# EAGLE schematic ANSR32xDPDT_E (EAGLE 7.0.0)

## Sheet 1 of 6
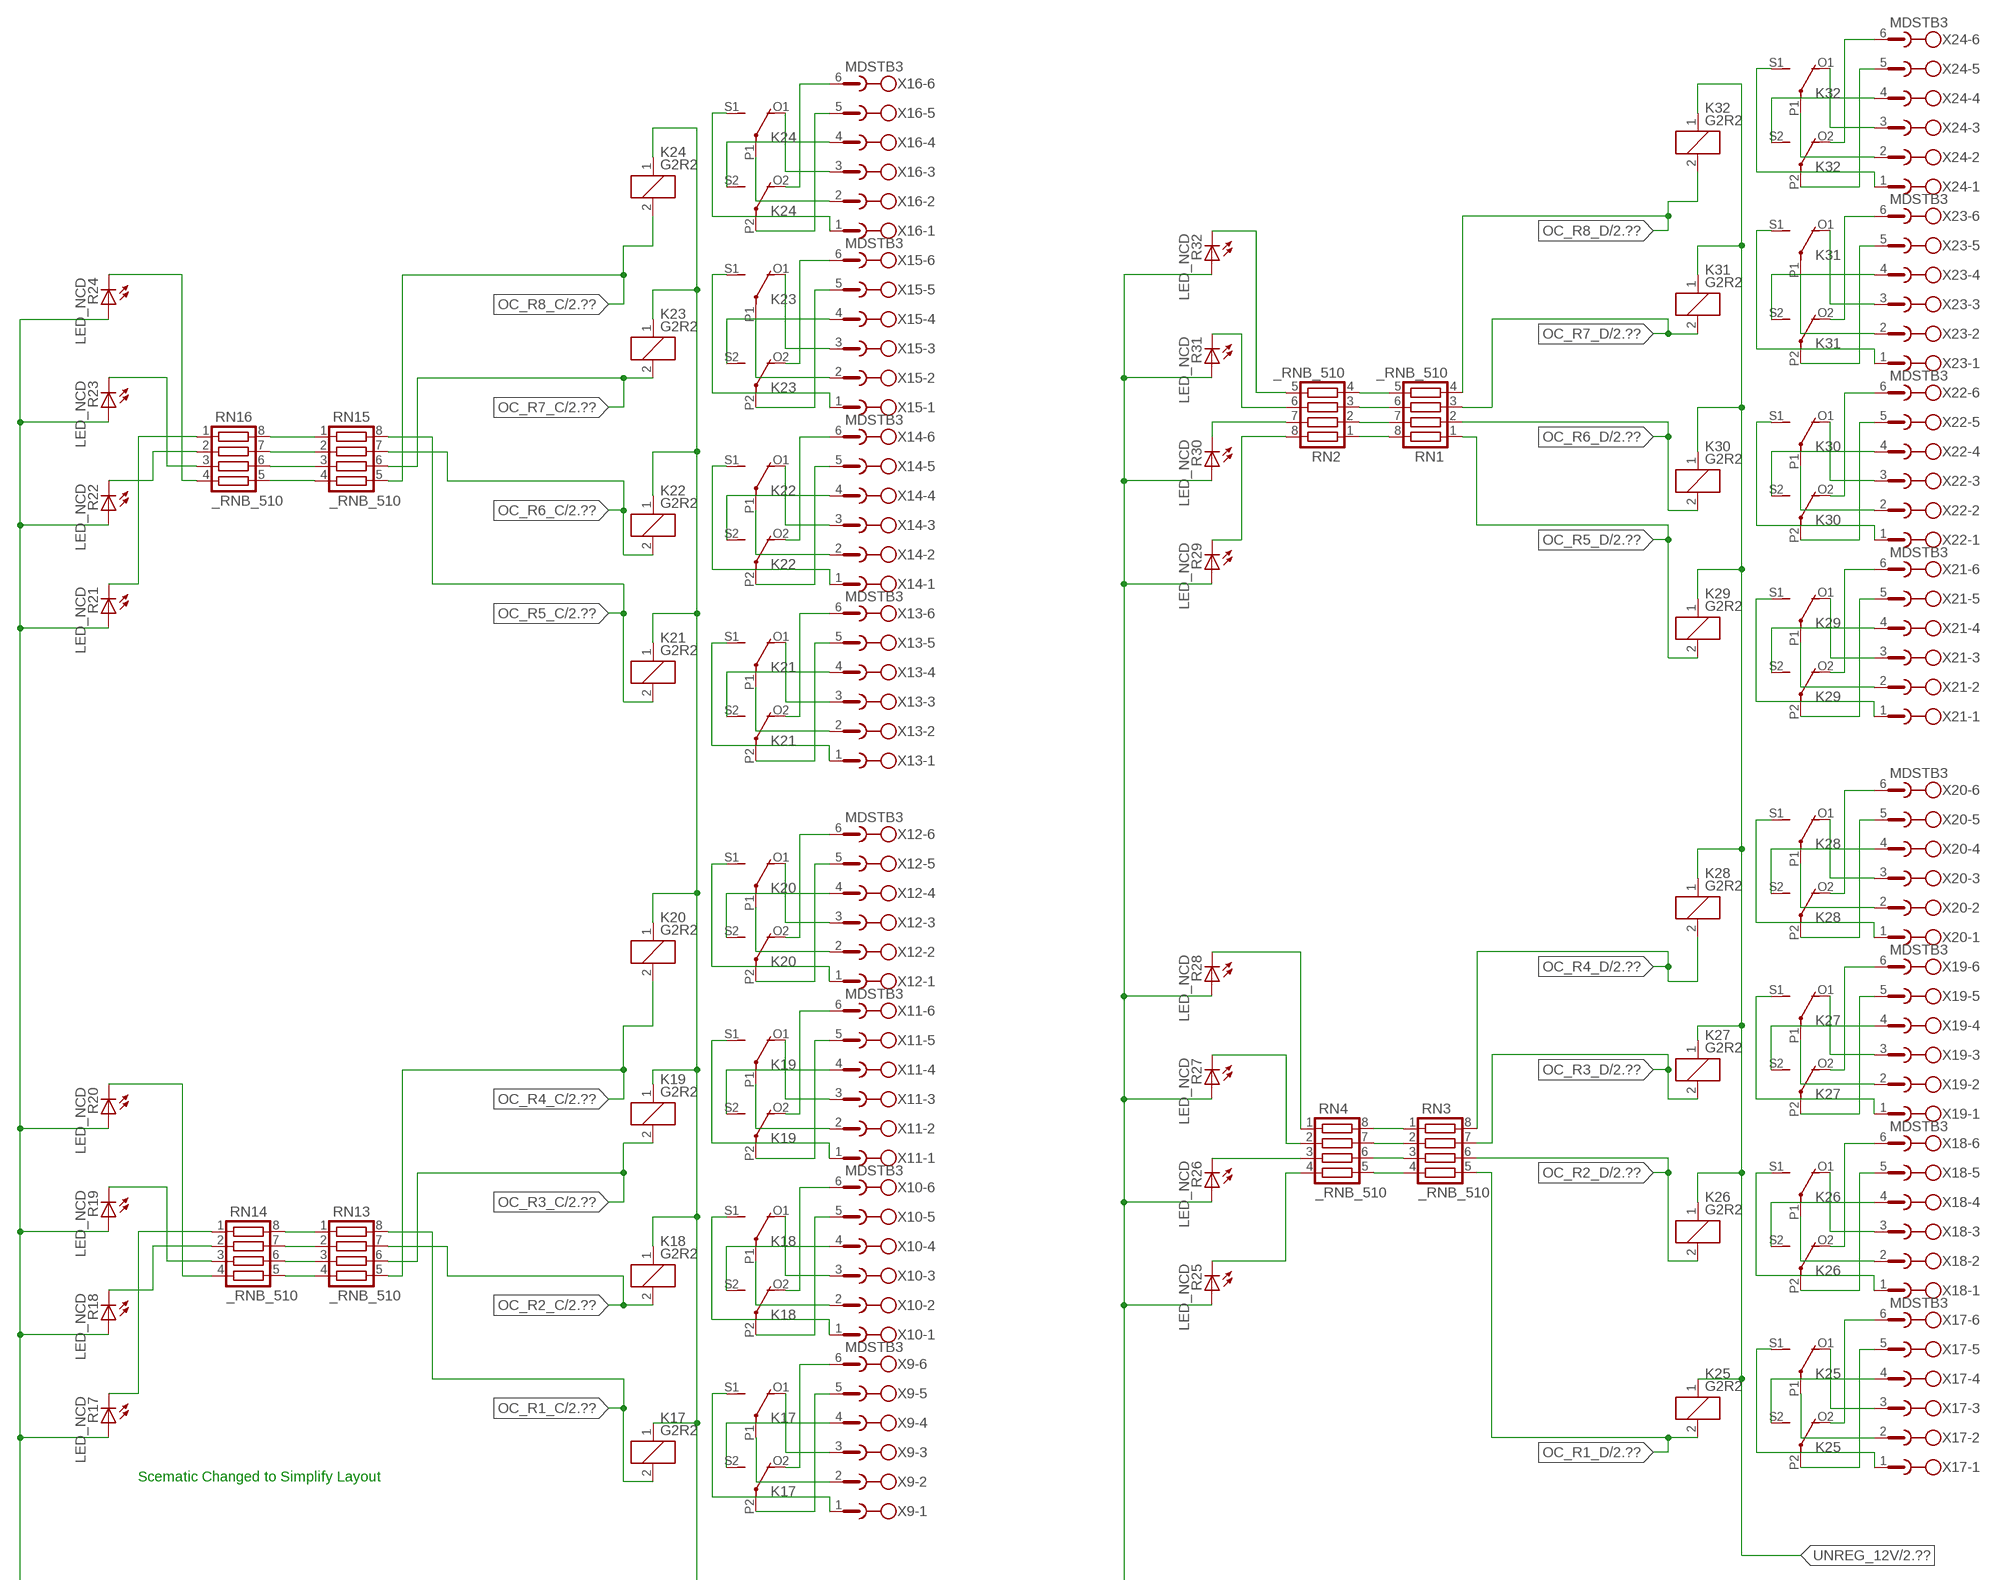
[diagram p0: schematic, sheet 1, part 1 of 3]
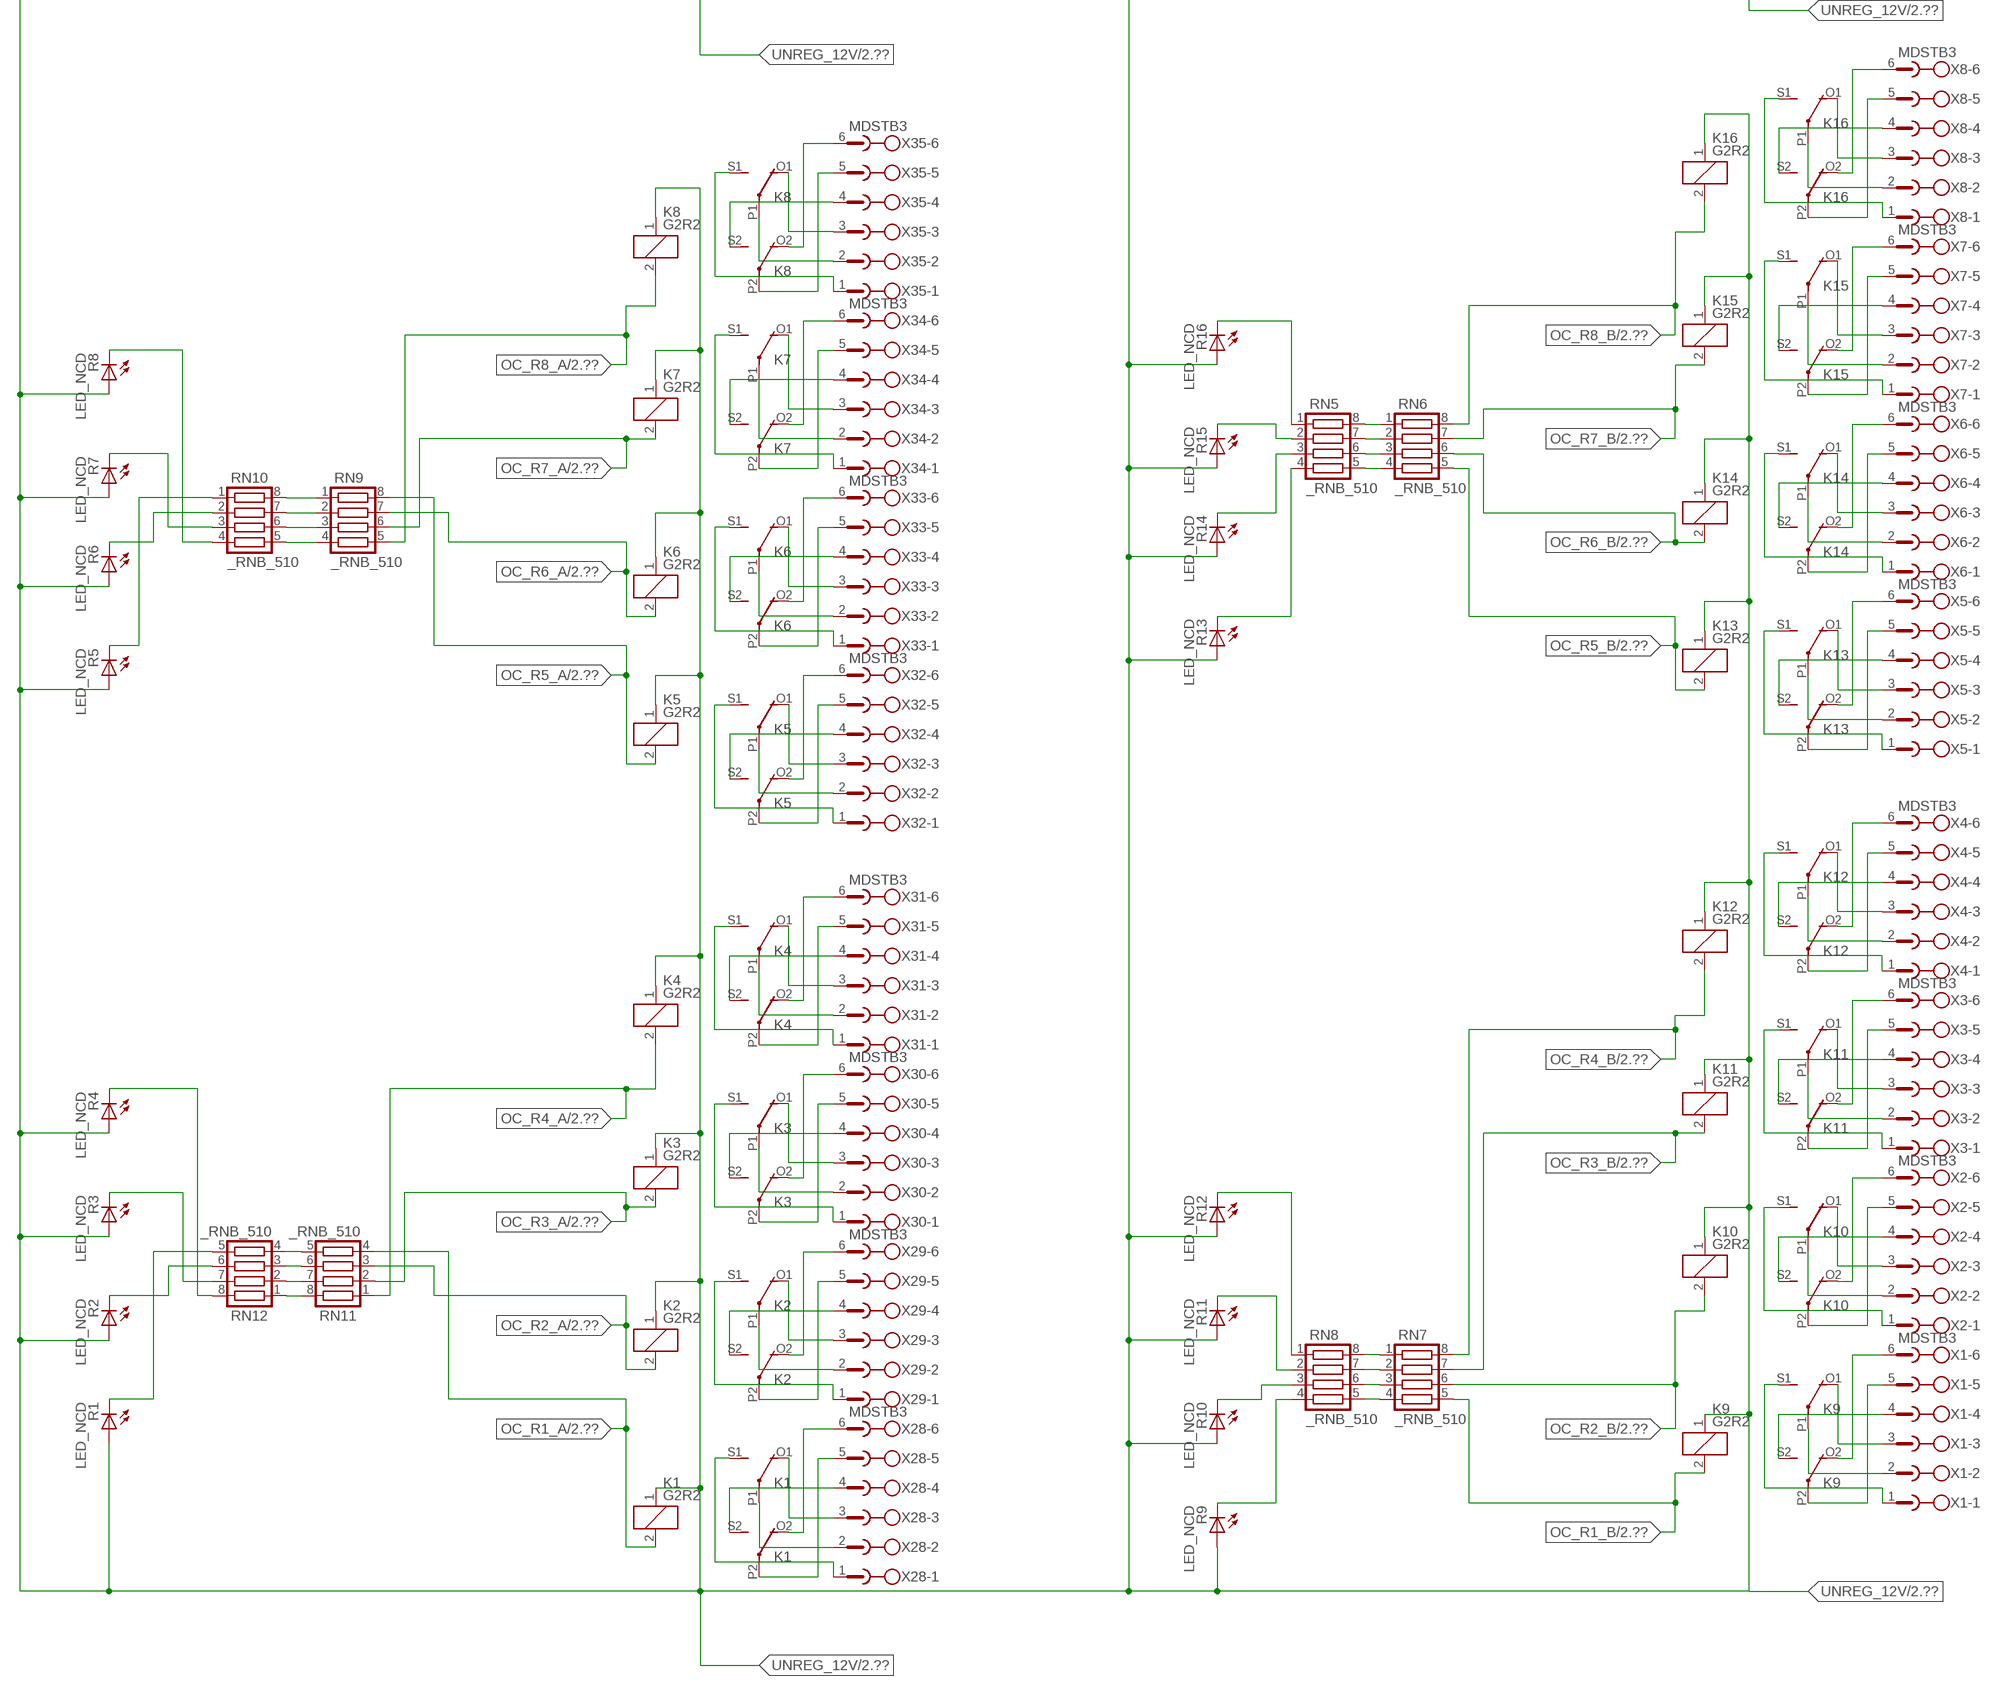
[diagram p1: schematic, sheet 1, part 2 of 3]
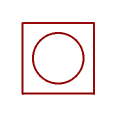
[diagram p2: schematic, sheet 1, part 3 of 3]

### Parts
K1  G2R2  [G2R2]
K2  G2R2  [G2R2]
K3  G2R2  [G2R2]
K4  G2R2  [G2R2]
K5  G2R2  [G2R2]
K6  G2R2  [G2R2]
K7  G2R2  [G2R2]
K8  G2R2  [G2R2]
K9  G2R2  [G2R2]
K10  G2R2  [G2R2]
K11  G2R2  [G2R2]
K12  G2R2  [G2R2]
K13  G2R2  [G2R2]
K14  G2R2  [G2R2]
K15  G2R2  [G2R2]
K16  G2R2  [G2R2]
K17  G2R2  [G2R2]
K18  G2R2  [G2R2]
K19  G2R2  [G2R2]
K20  G2R2  [G2R2]
K21  G2R2  [G2R2]
K22  G2R2  [G2R2]
K23  G2R2  [G2R2]
K24  G2R2  [G2R2]
K25  G2R2  [G2R2]
K26  G2R2  [G2R2]
K27  G2R2  [G2R2]
K28  G2R2  [G2R2]
K29  G2R2  [G2R2]
K30  G2R2  [G2R2]
K31  G2R2  [G2R2]
K32  G2R2  [G2R2]
R1  LED_NCD  [CHIPLED_0603]
R2  LED_NCD  [CHIPLED_0603]
R3  LED_NCD  [CHIPLED_0603]
R4  LED_NCD  [CHIPLED_0603]
R5  LED_NCD  [CHIPLED_0603]
R6  LED_NCD  [CHIPLED_0603]
R7  LED_NCD  [CHIPLED_0603]
R8  LED_NCD  [CHIPLED_0603]
R9  LED_NCD  [CHIPLED_0603]
R10  LED_NCD  [CHIPLED_0603]
R11  LED_NCD  [CHIPLED_0603]
R12  LED_NCD  [CHIPLED_0603]
R13  LED_NCD  [CHIPLED_0603]
R14  LED_NCD  [CHIPLED_0603]
R15  LED_NCD  [CHIPLED_0603]
R16  LED_NCD  [CHIPLED_0603]
R17  LED_NCD  [CHIPLED_0603]
R18  LED_NCD  [CHIPLED_0603]
R19  LED_NCD  [CHIPLED_0603]
R20  LED_NCD  [CHIPLED_0603]
R21  LED_NCD  [CHIPLED_0603]
R22  LED_NCD  [CHIPLED_0603]
R23  LED_NCD  [CHIPLED_0603]
R24  LED_NCD  [CHIPLED_0603]
R25  LED_NCD  [CHIPLED_0603]
R26  LED_NCD  [CHIPLED_0603]
R27  LED_NCD  [CHIPLED_0603]
R28  LED_NCD  [CHIPLED_0603]
R29  LED_NCD  [CHIPLED_0603]
R30  LED_NCD  [CHIPLED_0603]
R31  LED_NCD  [CHIPLED_0603]
R32  LED_NCD  [CHIPLED_0603]
RN1  _RNB_510  [RNB]
RN2  _RNB_510  [RNB]
RN3  _RNB_510  [RNB]
RN4  _RNB_510  [RNB]
RN5  _RNB_510  [RNB]
RN6  _RNB_510  [RNB]
RN7  _RNB_510  [RNB]
RN8  _RNB_510  [RNB]
RN9  _RNB_510  [RNB]
RN10  _RNB_510  [RNB]
RN11  _RNB_510  [RNB]
RN12  _RNB_510  [RNB]
RN13  _RNB_510  [RNB]
RN14  _RNB_510  [RNB]
RN15  _RNB_510  [RNB]
RN16  _RNB_510  [RNB]
U$1  PCB_MOUNTING_HOLE  [PCB_MOUNTING_HOLE]
X1  MDSTB3  [MDSTB3]
X2  MDSTB3  [MDSTB3]
X3  MDSTB3  [MDSTB3]
X4  MDSTB3  [MDSTB3]
X5  MDSTB3  [MDSTB3]
X6  MDSTB3  [MDSTB3]
X7  MDSTB3  [MDSTB3]
X8  MDSTB3  [MDSTB3]
X9  MDSTB3  [MDSTB3]
X10  MDSTB3  [MDSTB3]
X11  MDSTB3  [MDSTB3]
X12  MDSTB3  [MDSTB3]
X13  MDSTB3  [MDSTB3]
X14  MDSTB3  [MDSTB3]
X15  MDSTB3  [MDSTB3]
X16  MDSTB3  [MDSTB3]
X17  MDSTB3  [MDSTB3]
X18  MDSTB3  [MDSTB3]
X19  MDSTB3  [MDSTB3]
X20  MDSTB3  [MDSTB3]
X21  MDSTB3  [MDSTB3]
X22  MDSTB3  [MDSTB3]
X23  MDSTB3  [MDSTB3]
X24  MDSTB3  [MDSTB3]
X28  MDSTB3  [MDSTB3]
X29  MDSTB3  [MDSTB3]
X30  MDSTB3  [MDSTB3]
X31  MDSTB3  [MDSTB3]
X32  MDSTB3  [MDSTB3]
X33  MDSTB3  [MDSTB3]
X34  MDSTB3  [MDSTB3]
X35  MDSTB3  [MDSTB3]

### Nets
N$1: K9.P2(3:COM) X1.5
N$2: K9.O2(3:NC) X1.6
N$3: K9.S2(3:NO) X1.4
N$4: K9.P1(2:COM) X1.2
N$5: K9.O1(2:NC) X1.3
N$6: K9.S1(2:NO) X1.1
N$7: K10.P2(3:COM) X2.5
N$8: K10.O2(3:NC) X2.6
N$9: K10.S2(3:NO) X2.4
N$10: K10.S1(2:NO) X2.1
N$11: K10.P1(2:COM) X2.2
N$12: K10.O1(2:NC) X2.3
N$13: K11.P2(3:COM) X3.5
N$14: K11.O2(3:NC) X3.6
N$15: K12.P2(3:COM) X4.5
N$16: K12.O2(3:NC) X4.6
N$17: K11.S2(3:NO) X3.4
N$18: K12.S2(3:NO) X4.4
N$19: K11.O1(2:NC) X3.3
N$20: K12.O1(2:NC) X4.3
N$21: K12.P1(2:COM) X4.2
N$22: K11.P1(2:COM) X3.2
N$23: K11.S1(2:NO) X3.1
N$24: K12.S1(2:NO) X4.1
N$25: K13.O2(3:NC) X5.6
N$26: K13.P2(3:COM) X5.5
N$27: K13.S2(3:NO) X5.4
N$28: K13.P1(2:COM) X5.2
N$29: K13.S1(2:NO) X5.1
N$30: K13.O1(2:NC) X5.3
N$31: K14.P2(3:COM) X6.5
N$32: K14.O2(3:NC) X6.6
N$33: K14.P1(2:COM) X6.2
N$34: K14.S1(2:NO) X6.1
N$35: K15.P1(2:COM) X7.2
N$36: K16.P1(2:COM) X8.2
N$37: K16.P2(3:COM) X8.5
N$38: K16.O2(3:NC) X8.6
N$39: K14.O1(2:NC) X6.3
N$40: K16.O1(2:NC) X8.3
N$41: K15.O1(2:NC) X7.3
N$42: K15.O2(3:NC) X7.6
N$43: K15.P2(3:COM) X7.5
N$44: K14.S2(3:NO) X6.4
N$45: K15.S2(3:NO) X7.4
N$46: K15.S1(2:NO) X7.1
N$47: K16.S1(2:NO) X8.1
N$48: K16.S2(3:NO) X8.4
N$49: K17.P2(3:COM) X9.5
N$50: K17.O2(3:NC) X9.6
N$51: K17.S2(3:NO) X9.4
N$52: K17.P1(2:COM) X9.2
N$53: K17.O1(2:NC) X9.3
N$54: K17.S1(2:NO) X9.1
N$55: K18.P2(3:COM) X10.5
N$56: K18.O2(3:NC) X10.6
N$57: K18.S2(3:NO) X10.4
N$58: K18.S1(2:NO) X10.1
N$59: K18.P1(2:COM) X10.2
N$60: K18.O1(2:NC) X10.3
N$61: K19.P2(3:COM) X11.5
N$62: K19.O2(3:NC) X11.6
N$63: K20.P2(3:COM) X12.5
N$64: K20.O2(3:NC) X12.6
N$65: K19.S2(3:NO) X11.4
N$66: K20.S2(3:NO) X12.4
N$67: K19.O1(2:NC) X11.3
N$68: K20.O1(2:NC) X12.3
N$69: K20.P1(2:COM) X12.2
N$70: K19.P1(2:COM) X11.2
N$71: K19.S1(2:NO) X11.1
N$72: K20.S1(2:NO) X12.1
N$73: K21.O2(3:NC) X13.6
N$74: K21.P2(3:COM) X13.5
N$75: K21.S2(3:NO) X13.4
N$76: K21.P1(2:COM) X13.2
N$77: K21.S1(2:NO) X13.1
N$78: K21.O1(2:NC) X13.3
N$79: K22.P2(3:COM) X14.5
N$80: K22.O2(3:NC) X14.6
N$81: K22.P1(2:COM) X14.2
N$82: K22.S1(2:NO) X14.1
N$83: K23.P1(2:COM) X15.2
N$84: K24.P1(2:COM) X16.2
N$85: K24.P2(3:COM) X16.5
N$86: K24.O2(3:NC) X16.6
N$87: K22.O1(2:NC) X14.3
N$88: K24.O1(2:NC) X16.3
N$89: K23.O1(2:NC) X15.3
N$90: K23.O2(3:NC) X15.6
N$91: K23.P2(3:COM) X15.5
N$92: K22.S2(3:NO) X14.4
N$93: K23.S2(3:NO) X15.4
N$94: K23.S1(2:NO) X15.1
N$95: K24.S1(2:NO) X16.1
N$96: K24.S2(3:NO) X16.4
N$97: K25.P2(3:COM) X17.5
N$98: K25.O2(3:NC) X17.6
N$99: K25.S2(3:NO) X17.4
N$100: K25.P1(2:COM) X17.2
N$101: K25.O1(2:NC) X17.3
N$102: K25.S1(2:NO) X17.1
N$103: K26.P2(3:COM) X18.5
N$104: K26.O2(3:NC) X18.6
N$105: K26.S2(3:NO) X18.4
N$106: K26.S1(2:NO) X18.1
N$107: K26.P1(2:COM) X18.2
N$108: K26.O1(2:NC) X18.3
N$109: K27.P2(3:COM) X19.5
N$110: K27.O2(3:NC) X19.6
N$111: K28.P2(3:COM) X20.5
N$112: K28.O2(3:NC) X20.6
N$113: K27.S2(3:NO) X19.4
N$114: K28.S2(3:NO) X20.4
N$115: K27.O1(2:NC) X19.3
N$116: K28.O1(2:NC) X20.3
N$117: K28.P1(2:COM) X20.2
N$118: K27.P1(2:COM) X19.2
N$119: K27.S1(2:NO) X19.1
N$120: K28.S1(2:NO) X20.1
N$121: K29.O2(3:NC) X21.6
N$122: K29.P2(3:COM) X21.5
N$123: K29.S2(3:NO) X21.4
N$124: K29.P1(2:COM) X21.2
N$125: K29.S1(2:NO) X21.1
N$126: K29.O1(2:NC) X21.3
N$127: K30.P2(3:COM) X22.5
N$128: K30.O2(3:NC) X22.6
N$129: K30.P1(2:COM) X22.2
N$130: K30.S1(2:NO) X22.1
N$131: K31.P1(2:COM) X23.2
N$132: K32.P1(2:COM) X24.2
N$133: K32.P2(3:COM) X24.5
N$134: K32.O2(3:NC) X24.6
N$135: K30.O1(2:NC) X22.3
N$136: K32.O1(2:NC) X24.3
N$137: K31.O1(2:NC) X23.3
N$138: K31.O2(3:NC) X23.6
N$139: K31.P2(3:COM) X23.5
N$140: K30.S2(3:NO) X22.4
N$141: K31.S2(3:NO) X23.4
N$142: K31.S1(2:NO) X23.1
N$143: K32.S1(2:NO) X24.1
N$144: K32.S2(3:NO) X24.4
N$203: K1.P2(3:COM) X28.5
N$204: K1.O2(3:NC) X28.6
N$205: K1.S2(3:NO) X28.4
N$206: K1.P1(2:COM) X28.2
N$207: K1.O1(2:NC) X28.3
N$208: K1.S1(2:NO) X28.1
N$209: K2.P2(3:COM) X29.5
N$210: K2.O2(3:NC) X29.6
N$211: K2.S2(3:NO) X29.4
N$212: K2.S1(2:NO) X29.1
N$213: K2.P1(2:COM) X29.2
N$214: K2.O1(2:NC) X29.3
N$215: K3.P2(3:COM) X30.5
N$216: K3.O2(3:NC) X30.6
N$217: K4.P2(3:COM) X31.5
N$218: K4.O2(3:NC) X31.6
N$219: K3.S2(3:NO) X30.4
N$220: K4.S2(3:NO) X31.4
N$221: K3.O1(2:NC) X30.3
N$222: K4.O1(2:NC) X31.3
N$223: K4.P1(2:COM) X31.2
N$224: K3.P1(2:COM) X30.2
N$225: K3.S1(2:NO) X30.1
N$226: K4.S1(2:NO) X31.1
N$304: K5.O2(3:NC) X32.6
N$305: K5.P2(3:COM) X32.5
N$306: K5.S2(3:NO) X32.4
N$307: K5.P1(2:COM) X32.2
N$308: K5.S1(2:NO) X32.1
N$309: K5.O1(2:NC) X32.3
N$310: K6.P2(3:COM) X33.5
N$311: K6.O2(3:NC) X33.6
N$312: K6.P1(2:COM) X33.2
N$313: K6.S1(2:NO) X33.1
N$314: K7.P1(2:COM) X34.2
N$315: K8.P1(2:COM) X35.2
N$316: K8.P2(3:COM) X35.5
N$317: K8.O2(3:NC) X35.6
N$318: K6.O1(2:NC) X33.3
N$319: K8.O1(2:NC) X35.3
N$320: K7.O1(2:NC) X34.3
N$321: K7.O2(3:NC) X34.6
N$322: K7.P2(3:COM) X34.5
N$323: K6.S2(3:NO) X33.4
N$324: K7.S2(3:NO) X34.4
N$325: K7.S1(2:NO) X34.1
N$326: K8.S1(2:NO) X35.1
N$327: K8.S2(3:NO) X35.4
N$440: R30.C RN2.7
N$441: R16.C RN5.1
N$442: RN7.2 RN8.7
N$443: RN7.3 RN8.6
N$444: RN7.4 RN8.5
N$445: R15.C RN5.2
N$446: R26.C RN4.3
N$447: R13.C RN5.4
N$448: RN5.5 RN6.4
N$449: RN7.1 RN8.8
N$450: R12.C RN8.1
N$451: RN5.6 RN6.3
N$452: R11.C RN8.2
N$453: RN5.7 RN6.2
N$454: RN5.8 RN6.1
N$455: RN3.4 RN4.5
N$456: R32.C RN2.5
N$458: R14.C RN5.3
N$459: R10.C RN8.3
N$460: R29.C RN2.8
N$461: R28.C RN4.1
N$462: R27.C RN4.2
N$463: RN11.5 RN12.4
N$464: R25.C RN4.4
N$465: RN1.8 RN2.1
N$466: RN1.7 RN2.2
N$467: RN1.6 RN2.3
N$468: RN1.5 RN2.4
N$469: R31.C RN2.6
N$470: R9.C RN8.4
N$473: R1.C RN12.5
N$474: RN11.6 RN12.3
N$475: R2.C RN12.6
N$476: R3.C RN12.7
N$477: RN9.4 RN10.5
N$478: RN9.3 RN10.6
N$479: RN9.2 RN10.7
N$480: RN9.1 RN10.8
N$481: RN11.7 RN12.2
N$482: R5.C RN10.1
N$483: R4.C RN12.8
N$484: R7.C RN10.3
N$485: R8.C RN10.4
N$486: R6.C RN10.2
N$487: R19.C RN14.3
N$488: R18.C RN14.2
N$489: R17.C RN14.1
N$490: R24.C RN16.4
N$491: RN15.3 RN16.6
N$492: RN15.2 RN16.7
N$493: RN15.1 RN16.8
N$494: R20.C RN14.4
N$495: R23.C RN16.3
N$496: R22.C RN16.2
N$497: R21.C RN16.1
N$500: RN11.8 RN12.1
N$501: RN13.4 RN14.5
N$502: RN13.3 RN14.6
N$503: RN13.2 RN14.7
N$504: RN13.1 RN14.8
N$505: RN3.3 RN4.6
N$506: RN3.2 RN4.7
N$507: RN3.1 RN4.8
N$514: RN15.4 RN16.5
OC_R1_A: K1.2(1:C2) RN11.4 ; also sheet 2
OC_R1_B: K9.2(1:C2) RN7.5 ; also sheet 2
OC_R1_C: K17.2(1:C2) RN13.8 ; also sheet 2
OC_R1_D: K25.2(1:C2) RN3.5 ; also sheet 2
OC_R2_A: K2.2(1:C2) RN11.3 ; also sheet 2
OC_R2_B: K10.2(1:C2) RN7.6 ; also sheet 2
OC_R2_C: K18.2(1:C2) RN13.7 ; also sheet 2
OC_R2_D: K26.2(1:C2) RN3.6 ; also sheet 2
OC_R3_A: K3.2(1:C2) RN11.2 ; also sheet 2
OC_R3_B: K11.2(1:C2) RN7.7 ; also sheet 2
OC_R3_C: K19.2(1:C2) RN13.6 ; also sheet 2
OC_R3_D: K27.2(1:C2) RN3.7 ; also sheet 2
OC_R4_A: K4.2(1:C2) RN11.1 ; also sheet 2
OC_R4_B: K12.2(1:C2) RN7.8 ; also sheet 2
OC_R4_C: K20.2(1:C2) RN13.5 ; also sheet 2
OC_R4_D: K28.2(1:C2) RN3.8 ; also sheet 2
OC_R5_A: K5.2(1:C2) RN9.8 ; also sheet 2
OC_R5_B: K13.2(1:C2) RN6.5 ; also sheet 2
OC_R5_C: K21.2(1:C2) RN15.8 ; also sheet 2
OC_R5_D: K29.2(1:C2) RN1.1 ; also sheet 2
OC_R6_A: K6.2(1:C2) RN9.7 ; also sheet 2
OC_R6_B: K14.2(1:C2) RN6.6 ; also sheet 2
OC_R6_C: K22.2(1:C2) RN15.7 ; also sheet 2
OC_R6_D: K30.2(1:C2) RN1.2 ; also sheet 2
OC_R7_A: K7.2(1:C2) RN9.6 ; also sheet 2
OC_R7_B: K15.2(1:C2) RN6.7 ; also sheet 2
OC_R7_C: K23.2(1:C2) RN15.6 ; also sheet 2
OC_R7_D: K31.2(1:C2) RN1.3 ; also sheet 2
OC_R8_A: K8.2(1:C2) RN9.5 ; also sheet 2
OC_R8_B: K16.2(1:C2) RN6.8 ; also sheet 2
OC_R8_C: K24.2(1:C2) RN15.5 ; also sheet 2
OC_R8_D: K32.2(1:C2) RN1.4 ; also sheet 2
UNREG_12V: K1.1(1:C1) K2.1(1:C1) K3.1(1:C1) K4.1(1:C1) K5.1(1:C1) K6.1(1:C1) K7.1(1:C1) K8.1(1:C1) K9.1(1:C1) K10.1(1:C1) K11.1(1:C1) K12.1(1:C1) K13.1(1:C1) K14.1(1:C1) K15.1(1:C1) K16.1(1:C1) K17.1(1:C1) K18.1(1:C1) K19.1(1:C1) K20.1(1:C1) K21.1(1:C1) K22.1(1:C1) K23.1(1:C1) K24.1(1:C1) K25.1(1:C1) K26.1(1:C1) K27.1(1:C1) K28.1(1:C1) K29.1(1:C1) K30.1(1:C1) K31.1(1:C1) K32.1(1:C1) R1.A R2.A R3.A R4.A R5.A R6.A R7.A R8.A R9.A R10.A R11.A R12.A R13.A R14.A R15.A R16.A R17.A R18.A R19.A R20.A R21.A R22.A R23.A R24.A R25.A R26.A R27.A R28.A R29.A R30.A R31.A R32.A ; also sheet 2,3

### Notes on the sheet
- Scematic Changed to Simplify Layout

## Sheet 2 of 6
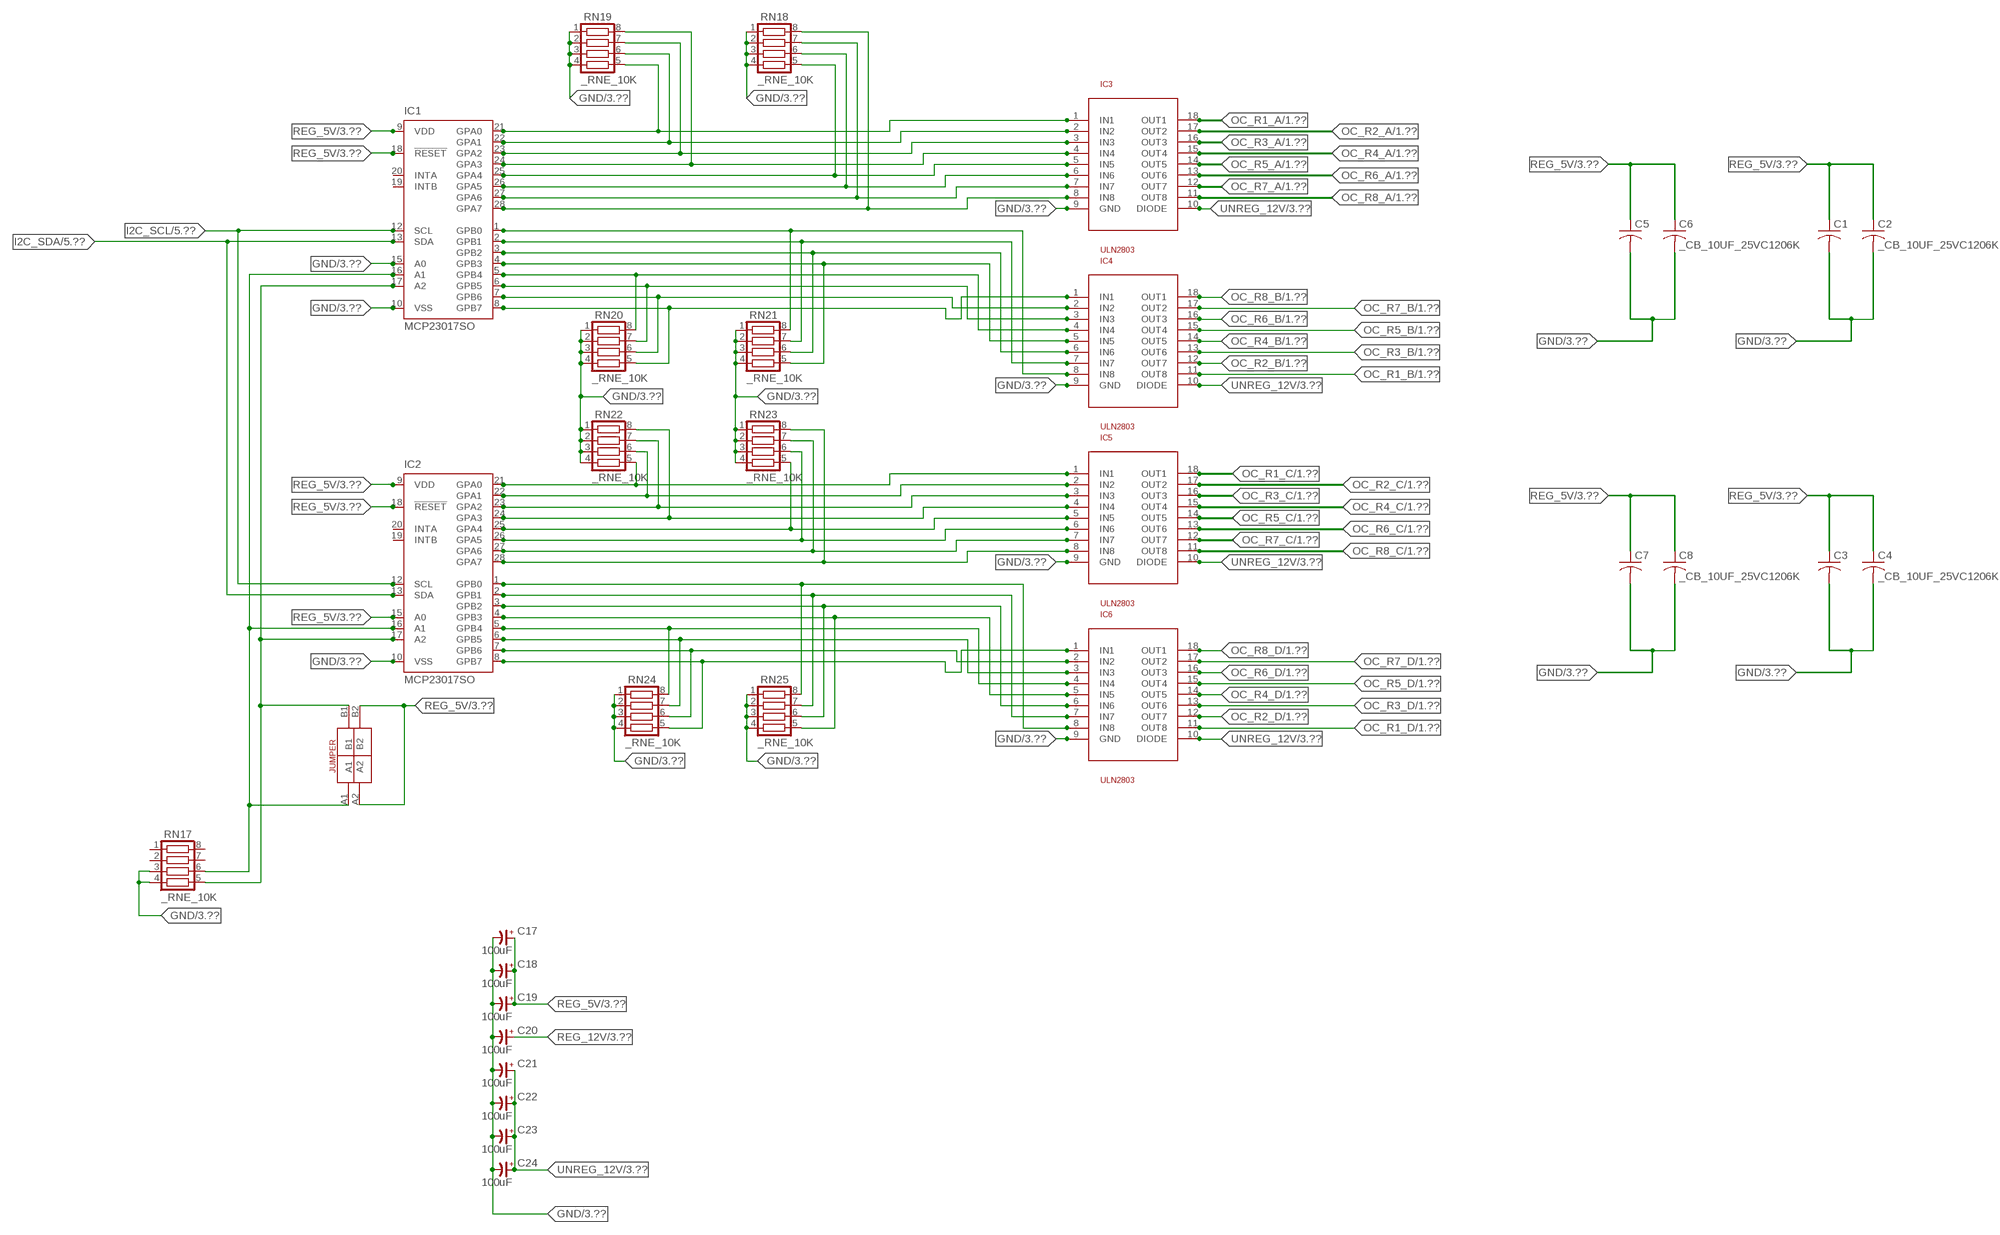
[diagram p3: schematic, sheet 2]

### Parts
C1  _CA_.10UF_50VC1206K  [_CA_.1UF_50V]
C2  _CB_10UF_25VC1206K  [_CB_10UF_25V]
C3  _CA_.10UF_50VC1206K  [_CA_.1UF_50V]
C4  _CB_10UF_25VC1206K  [_CB_10UF_25V]
C5  _CA_.10UF_50VC1206K  [_CA_.1UF_50V]
C6  _CB_10UF_25VC1206K  [_CB_10UF_25V]
C7  _CA_.10UF_50VC1206K  [_CA_.1UF_50V]
C8  _CB_10UF_25VC1206K  [_CB_10UF_25V]
C17  100uF  CP-E-025X060  [E-025X060]
C18  100uF  CP-E-025X060  [E-025X060]
C19  100uF  CP-E-025X060  [E-025X060]
C20  100uF  CP-E-025X060  [E-025X060]
C21  100uF  CP-E-025X060  [E-025X060]
C22  100uF  CP-E-025X060  [E-025X060]
C23  100uF  CP-E-025X060  [E-025X060]
C24  100uF  CP-E-025X060  [E-025X060]
IC1  MCP23017SO  [SO28W]
IC2  MCP23017SO  [SO28W]
IC3  ULN2803  [SO18L]
IC4  ULN2803  [SO18L]
IC5  ULN2803  [SO18L]
IC6  ULN2803  [SO18L]
RN17  _RNE_10K  [RNE]
RN18  _RNE_10K  [RNE]
RN19  _RNE_10K  [RNE]
RN20  _RNE_10K  [RNE]
RN21  _RNE_10K  [RNE]
RN22  _RNE_10K  [RNE]
RN23  _RNE_10K  [RNE]
RN24  _RNE_10K  [RNE]
RN25  _RNE_10K  [RNE]
U$13  JUMPER_2X2  [JUMPER_2X2]

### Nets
GND: C1.2 C2.2 C3.2 C4.2 C5.2 C6.2 C7.2 C8.2 C17.- C18.- C19.- C20.- C21.- C22.- C23.- C24.- IC1.10(VSS) IC1.15(A0) IC2.10(VSS) IC3.9(GND) IC4.9(GND) IC5.9(GND) IC6.9(GND) RN17.3 RN17.4 RN18.1 RN18.2 RN18.3 RN18.4 RN19.1 RN19.2 RN19.3 RN19.4 RN20.1 RN20.2 RN20.3 RN20.4 RN21.1 RN21.2 RN21.3 RN21.4 RN22.1 RN22.2 RN22.3 RN22.4 RN23.1 RN23.2 RN23.3 RN23.4 RN24.1 RN24.2 RN24.3 RN24.4 RN25.1 RN25.2 RN25.3 RN25.4 ; also sheet 3,4,5,6
I2C_SCL: IC1.12(SCL) IC2.12(SCL) ; also sheet 5,6
I2C_SDA: IC1.13(SDA) IC2.13(SDA) ; also sheet 5,6
N$405: IC1.21(GPA0) IC3.1(IN1) RN19.5
N$406: IC1.25(GPA4) IC3.5(IN5) RN18.5
N$407: IC1.26(GPA5) IC3.6(IN6) RN18.6
N$408: IC1.16(A1) IC2.16(A1) RN17.6 U$13.A1
N$409: IC1.22(GPA1) IC3.2(IN2) RN19.6
N$410: IC1.23(GPA2) IC3.3(IN3) RN19.7
N$411: IC1.24(GPA3) IC3.4(IN4) RN19.8
N$416: IC1.1(GPB0) IC4.8(IN8) RN21.8
N$417: IC1.2(GPB1) IC4.7(IN7) RN21.7
N$418: IC1.3(GPB2) IC4.6(IN6) RN21.6
N$419: IC1.4(GPB3) IC4.5(IN5) RN21.5
N$420: IC1.5(GPB4) IC4.4(IN4) RN20.8
N$421: IC1.6(GPB5) IC4.3(IN3) RN20.7
N$422: IC1.7(GPB6) IC4.2(IN2) RN20.6
N$423: IC1.8(GPB7) IC4.1(IN1) RN20.5
N$424: IC2.21(GPA0) IC5.1(IN1) RN22.5
N$425: IC2.22(GPA1) IC5.2(IN2) RN22.6
N$426: IC2.23(GPA2) IC5.3(IN3) RN22.7
N$427: IC2.24(GPA3) IC5.4(IN4) RN22.8
N$428: IC2.25(GPA4) IC5.5(IN5) RN23.5
N$429: IC2.26(GPA5) IC5.6(IN6) RN23.6
N$430: IC2.27(GPA6) IC5.7(IN7) RN23.7
N$431: IC2.28(GPA7) IC5.8(IN8) RN23.8
N$432: IC2.1(GPB0) IC6.8(IN8) RN25.8
N$433: IC2.2(GPB1) IC6.7(IN7) RN25.7
N$434: IC2.3(GPB2) IC6.6(IN6) RN25.6
N$435: IC2.4(GPB3) IC6.5(IN5) RN25.5
N$436: IC2.5(GPB4) IC6.4(IN4) RN24.8
N$437: IC2.6(GPB5) IC6.3(IN3) RN24.7
N$438: IC2.7(GPB6) IC6.2(IN2) RN24.6
N$439: IC2.8(GPB7) IC6.1(IN1) RN24.5
N$498: IC1.17(A2) IC2.17(A2) RN17.5 U$13.B1
N$525: IC1.27(GPA6) IC3.7(IN7) RN18.7
N$526: IC1.28(GPA7) IC3.8(IN8) RN18.8
OC_R1_A: IC3.18(OUT1) ; also sheet 1
OC_R1_B: IC4.11(OUT8) ; also sheet 1
OC_R1_C: IC5.18(OUT1) ; also sheet 1
OC_R1_D: IC6.11(OUT8) ; also sheet 1
OC_R2_A: IC3.17(OUT2) ; also sheet 1
OC_R2_B: IC4.12(OUT7) ; also sheet 1
OC_R2_C: IC5.17(OUT2) ; also sheet 1
OC_R2_D: IC6.12(OUT7) ; also sheet 1
OC_R3_A: IC3.16(OUT3) ; also sheet 1
OC_R3_B: IC4.13(OUT6) ; also sheet 1
OC_R3_C: IC5.16(OUT3) ; also sheet 1
OC_R3_D: IC6.13(OUT6) ; also sheet 1
OC_R4_A: IC3.15(OUT4) ; also sheet 1
OC_R4_B: IC4.14(OUT5) ; also sheet 1
OC_R4_C: IC5.15(OUT4) ; also sheet 1
OC_R4_D: IC6.14(OUT5) ; also sheet 1
OC_R5_A: IC3.14(OUT5) ; also sheet 1
OC_R5_B: IC4.15(OUT4) ; also sheet 1
OC_R5_C: IC5.14(OUT5) ; also sheet 1
OC_R5_D: IC6.15(OUT4) ; also sheet 1
OC_R6_A: IC3.13(OUT6) ; also sheet 1
OC_R6_B: IC4.16(OUT3) ; also sheet 1
OC_R6_C: IC5.13(OUT6) ; also sheet 1
OC_R6_D: IC6.16(OUT3) ; also sheet 1
OC_R7_A: IC3.12(OUT7) ; also sheet 1
OC_R7_B: IC4.17(OUT2) ; also sheet 1
OC_R7_C: IC5.12(OUT7) ; also sheet 1
OC_R7_D: IC6.17(OUT2) ; also sheet 1
OC_R8_A: IC3.11(OUT8) ; also sheet 1
OC_R8_B: IC4.18(OUT1) ; also sheet 1
OC_R8_C: IC5.11(OUT8) ; also sheet 1
OC_R8_D: IC6.18(OUT1) ; also sheet 1
REG_5V: C1.1 C2.1 C3.1 C4.1 C5.1 C6.1 C7.1 C8.1 C17.+ C18.+ C19.+ IC1.9(VDD) IC1.18(!RESET) IC2.9(VDD) IC2.15(A0) IC2.18(!RESET) U$13.A2 U$13.B2 ; also sheet 3,4,5,6
REG_12V: C20.+ ; also sheet 3,4
UNREG_12V: C21.+ C22.+ C23.+ C24.+ IC3.10(DIODE) IC4.10(DIODE) IC5.10(DIODE) IC6.10(DIODE) ; also sheet 1,3
Unconnected: IC1.19(INTB) IC1.20(INTA) IC2.19(INTB) IC2.20(INTA) RN17.1 RN17.2 RN17.7 RN17.8

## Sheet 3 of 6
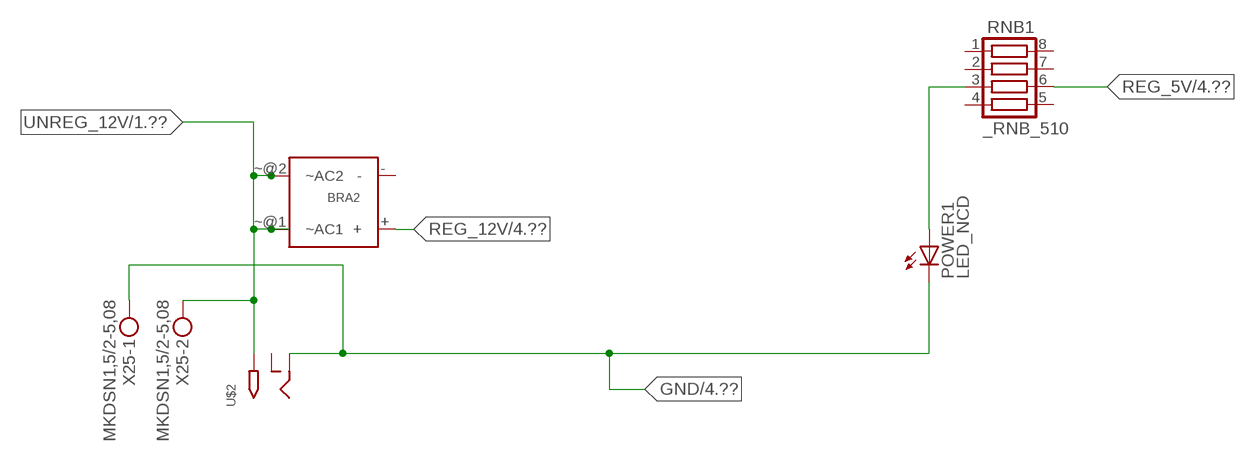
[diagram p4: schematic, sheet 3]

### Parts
BRA2  MB2S_  [MB2S]
POWER1  LED_NCD  [CHIPLED_0603]
RNB1  _RNB_510  [RNB]
U$2  2.1MMJACK  [PJ-102A]
X25  MKDSN1,5/2-5,08  [MKDSN1,5/2-5,08]

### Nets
GND: POWER1.C U$2.RING X25.1 ; also sheet 2,4,5,6
N$163: POWER1.A RNB1.3
REG_5V: RNB1.6 ; also sheet 2,4,5,6
REG_12V: BRA2.+ ; also sheet 2,4
UNREG_12V: BRA2.~@1(~AC1) BRA2.~@2(~AC2) U$2.TIP X25.2 ; also sheet 1,2
Unconnected: BRA2.- RNB1.1 RNB1.2 RNB1.4 RNB1.5 RNB1.7 RNB1.8 U$2.RING_SW

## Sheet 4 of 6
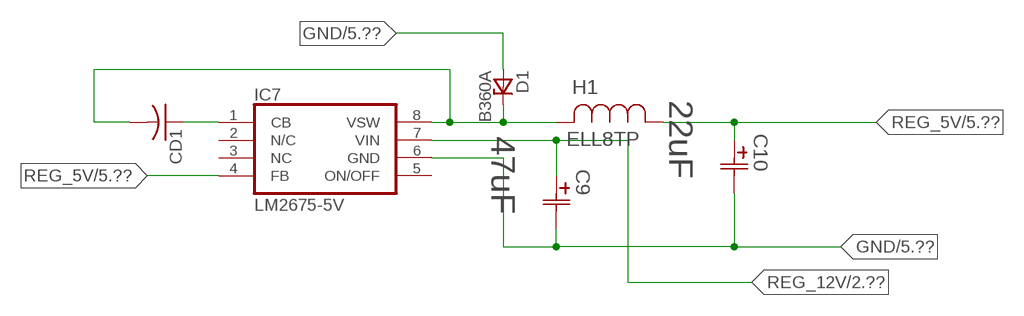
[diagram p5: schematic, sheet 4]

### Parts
C9  47uF  490-5463-6-NDCAP  [C2917(7343)-Y]
C10  22uF  490-5463-6-NDCAP  [C2917(7343)-Y]
CD1  _CD_10NF_50VC1206K  [_CD_10NF_50V]
D1  B360A  [DO214AC_ZENER]
H1  ELL8TP  [IND_ELL8TP]
IC7  LM2675-5V  LM2675  [SO-8]

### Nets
GND: C9.2(C2) C10.2(C2) D1.A IC7.6(GND) ; also sheet 2,3,5,6
N$164: CD1.2 D1.C H1.2 IC7.8(VSW)
N$165: CD1.1 IC7.1(CB)
REG_5V: C10.1(C1) H1.1 IC7.4(FB) ; also sheet 2,3,5,6
REG_12V: C9.1(C1) IC7.7(VIN) ; also sheet 2,3
Unconnected: IC7.2(N/C) IC7.5(ON/OFF)

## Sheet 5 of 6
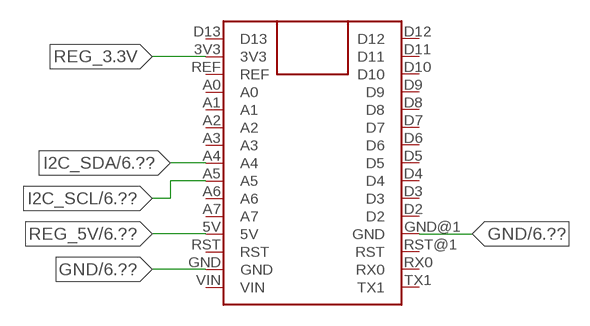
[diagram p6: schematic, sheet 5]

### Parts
FOR_NANO  ARDUINO_NANO  [ARDUINO_NANO]

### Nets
GND: FOR_NANO.GND FOR_NANO.GND@1(GND) ; also sheet 2,3,4,6
I2C_SCL: FOR_NANO.A5 ; also sheet 2,6
I2C_SDA: FOR_NANO.A4 ; also sheet 2,6
REG_3.3V: FOR_NANO.3V3
REG_5V: FOR_NANO.5V ; also sheet 2,3,4,6
Unconnected: FOR_NANO.A0 FOR_NANO.A1 FOR_NANO.A2 FOR_NANO.A3 FOR_NANO.A6 FOR_NANO.A7 FOR_NANO.D2 FOR_NANO.D3 FOR_NANO.D4 FOR_NANO.D5 FOR_NANO.D6 FOR_NANO.D7 FOR_NANO.D8 FOR_NANO.D9 FOR_NANO.D10 FOR_NANO.D11 FOR_NANO.D12 FOR_NANO.D13 FOR_NANO.REF FOR_NANO.RST FOR_NANO.RST@1(RST) FOR_NANO.RX0 FOR_NANO.TX1 FOR_NANO.VIN

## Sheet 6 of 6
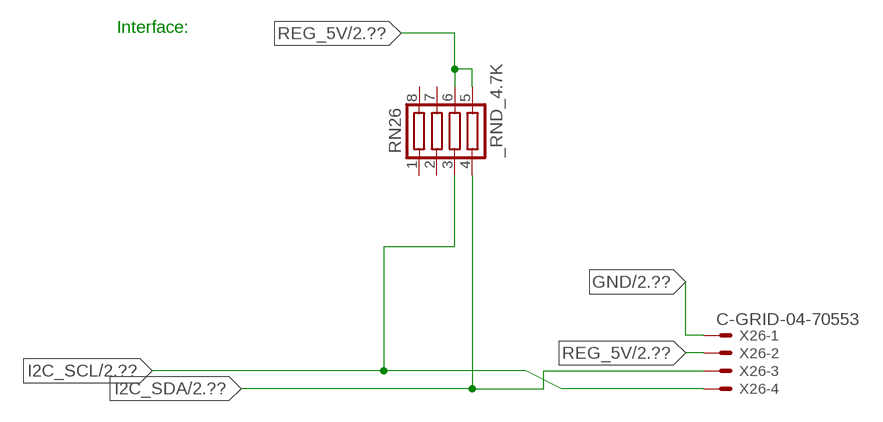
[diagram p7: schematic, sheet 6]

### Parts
RN26  _RND_4.7K  [RND]
X26  C-GRID-04-70553  [70553-04]

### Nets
GND: X26.1 ; also sheet 2,3,4,5
I2C_SCL: RN26.3 X26.4 ; also sheet 2,5
I2C_SDA: RN26.4 X26.3 ; also sheet 2,5
REG_5V: RN26.5 RN26.6 X26.2 ; also sheet 2,3,4,5
Unconnected: RN26.1 RN26.2 RN26.7 RN26.8

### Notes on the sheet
- Interface:

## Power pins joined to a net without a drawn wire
NC: IC7.3(NC)

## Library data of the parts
BRA2 = NCD_ULTIMATE_LIBRARY:MB2S: Bridge Rectifier BRA MB2S 200V 500ma Digikey MB2S-TPMSTR-ND/MB2S-TP
C1 C3 C5 C7 = NCD_ULTIMATE_LIBRARY:_CA_.10UF_50V: Capacitor .1uF SMT
C2 C4 C6 C8 = NCD_ULTIMATE_LIBRARY:_CB_10UF_25V: Capacitor 10uF SMT
C9 C10 = NCD_ULTIMATE_bhaskar:490-5463-6-ND: NCD CAP
C17-C24 = NCD_ULTIMATE_LIBRARY:CP-: Capacitors All Kinds POLARIZED CAP
CD1 = NCD_ULTIMATE_LIBRARY:_CD_10NF_50V: Capacitor 10nF SMT
D1 = NCD_ULTIMATE_bhaskar:B360A: NCD DIODE B350A/B360A
FOR_NANO = NCD_ULTIMATE_CONNECTORS:ARDUINO_NANO
H1 = NCD_ULTIMATE_bhaskar:ELL8TP: NCD coil
IC1 IC2 = NCD_ULTIMATE_LIBRARY:MCP23017: Semiconductor Port Expander I/O 16-Bit I2C http://ww1.microchip.com/downloads/en/DeviceDoc/21952a.pdf Source: http://ww1.microchip.com/downloads/en/DeviceDoc/21952a.pdf
IC3-IC6 = NCD_ULTIMATE_LIBRARY:ULN2803: Semiconductor 8 O.C. N-Channel Transistor Driver Digikey ULN2803AFWGCELTR-ND/ULN2803AFWG,C,EL
IC7 = NCD_ULTIMATE_bhaskar:LM2675: LM2675 NCD http://www.ti.com/lit/ds/symlink/lm2675.pdf
K1-K32 = NCD_ULTIMATE_LIBRARY:G2R2: RELAY 2 x switch, Omron
POWER1 R1-R32 = NCD_ULTIMATE_bhaskar:LED_NCD
RN1-RN16 RNB1 = NCD_ULTIMATE_LIBRARY:_RNB_510: Resistor Array RNB SMT 510 x 4 Single Resistor Source: http://www.ctscorp.com/components/Datasheets/CTSChipArrayDs.pdf Digikey 742C083511JPTR-ND/ 742C083511JP; OC_FARNELL: unknown; OC_NEWARK: unknown
RN17-RN25 = NCD_ULTIMATE_LIBRARY:_RNE_10K: Resistor Array RNE SMT 10K x 4 Single Resistor Source: http://www.ctscorp.com/components/Datasheets/CTSChipArrayDs.pdf Digikey 742C083103JPTR-ND/742C083103JP; OC_FARNELL: unknown; OC_NEWARK: unknown
RN26 = NCD_ULTIMATE_LIBRARY:_RND_4.7K: Resistor Array RND SMT 4.7K x 4 Single Resistor Source: http://www.ctscorp.com/components/Datasheets/CTSChipArrayDs.pdf Digikey 742C083472JPTR-ND/742C083472JP; OC_FARNELL: unknown; OC_NEWARK: unknown
U$1 = NCD_ULTIMATE_CONNECTORS:PCB_MOUNTING_HOLE
U$2 = NCD_ULTIMATE_CONNECTORS:2.1MMJACK: 2.1mm x 5.5mm DC jack with internal switch. Digikey part #PJ-102A, 4UCON part #05537 By microbuilder.eu
U$13 = NCD_ULTIMATE_CONNECTORS:JUMPER_2X2
X1-X24 X28-X35 = NCD_ULTIMATE_LIBRARY:MDSTB3: PHOENIX
X25 = NCD_ULTIMATE_CONNECTORS:MKDSN1,5/2-5,08: MKDSN 1,5/ 2-5,08 Printklemme
X26 = NCD_ULTIMATE_CONNECTORS:C-GRID-04: CONNECTOR 4-Pos I2C wire to board 2.54 mm (0.100") pitch header Digikey WM1342-ND/0015912045; OC_FARNELL: unknown; OC_NEWARK: unknown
